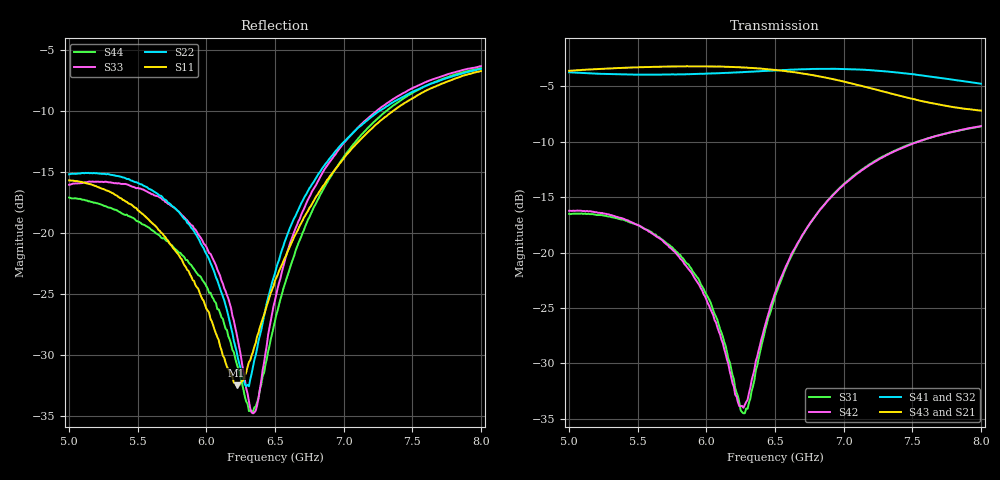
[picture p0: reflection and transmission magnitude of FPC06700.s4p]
# MHz S MA R 50
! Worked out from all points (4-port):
!   301 points, 5 GHz to 8 GHz, reference 50 ohm
!   strongest paths, dB at 5 GHz, 5.75 GHz, 6.5 GHz, 7.25 GHz, 8 GHz:
!     S43: -3.6, -3.2, -3.5, -5.3, -7.2
!     S21: -3.7, -3.2, -3.6, -5.3, -7.0
!     S41: -3.7, -3.9, -3.6, -3.6, -4.8
!     S32: -3.7, -4.0, -3.6, -3.7, -4.8
!     S42: -16.2, -19.7, -23.7, -11.6, -8.6
!     S31: -16.5, -19.5, -24.0, -11.6, -8.6
!   lowest |S11| = -32.5 dB at 6.22 GHz (marker M1), VSWR 1.05, Z = 49.8 + j2.37 ohm
!   |S11| at or under -10 dB: start of sweep to 7.36 GHz
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5000  0.1643 15.7  0.6561 105.0  0.1494 168.2  0.652 10.2
      0.6562 104.9  0.1741 -109.6  0.6493 128.2  0.1542 -74.1
      0.1496 168.2  0.6494 128.3  0.1577 -133.2  0.6623 -143.7
      0.6515 10.2  0.1544 -74.1  0.6615 -143.7  0.1398 -131.5
5670  0.1004 -98.5  0.6887 10.9  0.1149 86.6  0.6356 -83.6
      0.6886 10.9  0.1421 162.3  0.6296 51.0  0.1143 -141.8
      0.115 86.4  0.63 51.0  0.1392 149.7  0.6905 137.0
      0.6361 -83.6  0.1144 -141.7  0.6908 137.0  0.09582 152.5
6220  0.02379 92.5  0.6852 -67.6  0.02329 53.5  0.6505 -162.0
      0.6851 -67.6  0.03281 52.3  0.6512 -14.2  0.02217 -152.4
      0.02329 53.0  0.651 -14.2  0.03882 111.7  0.6874 70.9
      0.6503 -161.9  0.02235 -152.3  0.6871 71.0  0.0293 125.5
6360  0.03563 13.2  0.6767 -87.7  0.02924 116.3  0.6577 177.7
      0.6767 -87.7  0.0317 -47.8  0.658 -31.4  0.032 -92.9
      0.02928 116.5  0.6582 -31.4  0.0188 174.9  0.6799 53.9
      0.6573 177.7  0.03226 -92.8  0.6794 54.0  0.01953 178.2
6980  0.1951 -141.2  0.5931 -175.4  0.1981 56.7  0.6748 84.4
      0.5926 -175.4  0.2296 -174.8  0.6663 -110.2  0.1966 -139.4
      0.1983 56.8  0.6671 -110.2  0.226 173.3  0.5955 -20.5
      0.6747 84.4  0.1968 -139.5  0.5953 -20.5  0.1974 174.9
7480  0.3503 126.4  0.5059 119.3  0.3072 -16.3  0.6404 7.8
      0.5062 119.3  0.3736 120.3  0.6317 -174.2  0.3059 160.1
      0.3075 -16.2  0.6319 -174.3  0.3866 115.5  0.4976 -74.5
      0.6413 7.8  0.3059 160.0  0.4977 -74.6  0.3689 115.0
8000  0.4603 41.2  0.4467 56.5  0.3705 -87.9  0.5783 -69.0
      0.447 56.4  0.4702 60.4  0.5735 121.5  0.3722 100.8
      0.3709 -87.8  0.5734 121.5  0.4822 55.1  0.4374 -124.1
      0.5786 -69.0  0.372 100.8  0.4375 -124.1  0.4733 53.3
